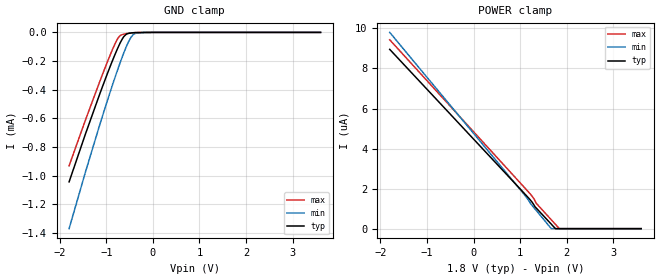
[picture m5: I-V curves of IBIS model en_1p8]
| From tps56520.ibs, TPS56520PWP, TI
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|   en_1p8 Model
[Model]   en_1p8
Model_type   Input
Vinl = 0.6
Vinh = 1.26
|   typ   min   max
|   (nom PVT)   (fast PVT)   (slow PVT)
C_comp   5.309e-12   4.968e-12   5.567e-12
| Where nom  PVT is Nominal Process, 1.8V, 27C
|   Fast PVT is Strong Process,  1.9V, -40C
|   Slow PVT is Weak Process,   1.7V, 125C
[Voltage Range]   1.8   1.7   1.9
|Junction Temperature
[Temperature Range]   27   125   -40
[Power Clamp Reference]   1.8   1.7   1.9
[GND Clamp Reference]   0   0   0
[GND Clamp]
|   Voltage   I(typ)   I(min)   I(max)
-1.8V     -1.044mA   -1.371mA   -931.7uA
-1.457V   -716.9uA   -983.9uA   -619.1uA
-1.135V   -423.9uA   -638.1uA   -337.4uA
-825.3mV  -162.9uA   -325.2uA   -87.9uA
-732.4mV  -93.38uA   -237.5uA   -32.27uA
-693.3mV  -67.06uA   -201.9uA   -19.95uA
-619.2mV  -27.12uA   -137.8uA   -11.71uA
-519.4mV  -6.693uA   -62.67uA   -5.912uA
-423mV    -2.599uA   -15.98uA   -2.336uA
-349.9mV  -1.346uA   -4.005uA   -1.246uA
-173.1mV  -527.4nA   -605.3nA   -577.6nA
3.6V      0A         0A         0A
[POWER Clamp]
|   Voltage   I(typ)   I(min)   I(max)
-1.8V     8.955uA    9.803uA    9.434uA
991.4mV   2.008uA    1.982uA    2.313uA
1.193V    1.501uA    1.374uA    1.796uA
1.286V    1.227uA    1.079uA    1.531uA
1.346V    1.028uA    909.3nA    1.268uA
1.67V     223.3nA    0A         442.6nA
1.759V    0A         0A         215.8nA
1.842V    0A         0A         0A
3.6V      0A         0A         0A
